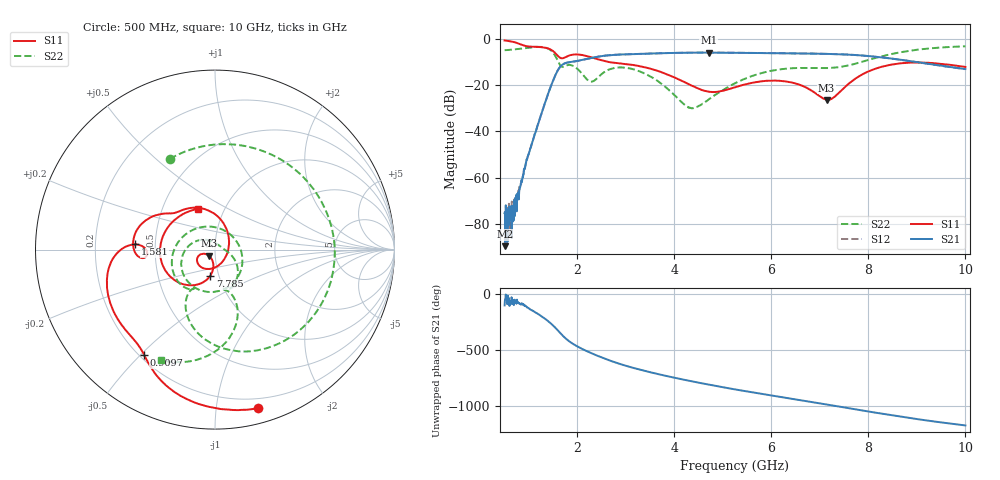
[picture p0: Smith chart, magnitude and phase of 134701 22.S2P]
!  2-Port S-parameters saved by WinCal
! VAR MeasName=S-Parameters (CALIBRATED_DATA) read from VNA (N5242A)
! VAR MeasDate=2013-7-3 16:31:38
! VAR NAME=134701 22
! VAR FILENAME=134701 22.S2P
! VAR DATE=2013-7-3 16:31:38
! VAR PHYS_PORTS=1,2
# Hz S MA R 50
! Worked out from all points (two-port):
!   1601 points, 500 MHz to 10 GHz, reference 50 ohm
!   highest |S21| = -5.98 dB at 4.71 GHz (marker M1); lowest = -89.5 dB at 517.8 MHz (marker M2)
!   |S21| within 3 dB of the highest: 2.137 GHz to 8.633 GHz (6.496 GHz wide, 121 % of centre)
!   lowest |S11| = -26.4 dB at 7.138 GHz (marker M3), VSWR 1.10, Z = 46.5 - j3.11 ohm
!   |S11| at or under -10 dB: 2.636 GHz to end of sweep
!   |S22| runs from -30.0 to -3.3 dB; largest |S21 - S12| = 0.0029
!   S11 on the Smith chart (normalised r, x): 500 MHz: 0.12, -1.30; 909.7 MHz: 0.22, -0.51; 1.581 GHz: 0.38, +0.03; 7.785 GHz: 0.91, -0.27; 10 GHz: 0.75, +0.36
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5e8  0.9168 -74.9  0.0001733 -105.1  0.0001792 -35.8  0.5645 116.6
5.178125e8  0.9117 -77.3  3.367e-05 -40.0  8.568e-05 16.9  0.5663 114.1
7.1375e8  0.8337 -104.0  0.0001516 -83.8  0.0003533 -77.5  0.5899 84.7
9.096875e8  0.7076 -124.0  0.001527 -109.4  0.001612 -106.4  0.6252 50.5
1.2125e9  0.6626 -147.6  0.0172 172.3  0.01733 172.1  0.6696 -15.7
1.4025e9  0.6127 -167.6  0.06755 112.7  0.06753 112.5  0.6078 -67.7
1.580625e9  0.4478 176.3  0.1943 40.3  0.1937 40.2  0.3613 -116.9
1.735e9  0.3912 -173.7  0.2929 -30.2  0.2923 -30.3  0.2539 -119.5
2.085312e9  0.4477 165.5  0.3462 -130.0  0.3454 -130.0  0.1814 150.5
2.453438e9  0.3524 145.6  0.414 159.1  0.4137 159.1  0.1557 -13.7
2.85125e9  0.2944 134.4  0.4538 96.6  0.453 96.5  0.2399 -103.3
3.670625e9  0.2 91.1  0.4847 2.2  0.4838 2.2  0.1195 157.9
4.305938e9  0.1036 42.6  0.4994 -57.1  0.4999 -57.0  0.03244 68.3
4.709688e9  0.07196 -8.1  0.5022 -91.2  0.502 -91.2  0.04934 3.8
5.25e9  0.0897 -76.9  0.4979 -133.6  0.4983 -133.6  0.1094 -23.3
6.004062e9  0.1248 -130.7  0.4877 171.6  0.4879 171.4  0.2039 -53.4
6.835312e9  0.07517 -161.7  0.4776 113.2  0.4774 113.2  0.2328 -75.8
7.138125e9  0.0481 -136.2  0.471 91.8  0.4706 91.6  0.2321 -75.8
7.785312e9  0.1497 -100.5  0.4408 45.1  0.441 44.9  0.2996 -68.3
8.420625e9  0.2693 -135.8  0.3798 -0.3  0.3793 -0.6  0.454 -76.3
9.16875e9  0.3044 175.1  0.2948 -48.4  0.2936 -48.9  0.6037 -96.0
1e10  0.2461 113.2  0.2216 -95.1  0.2202 -95.5  0.6855 -116.2
